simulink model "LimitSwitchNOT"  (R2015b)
settings: Solver=VariableStepAuto  StartTime=0.0  StopTime=10.0  RelTol=1e-3
libraries: vexarmcortexlib x4

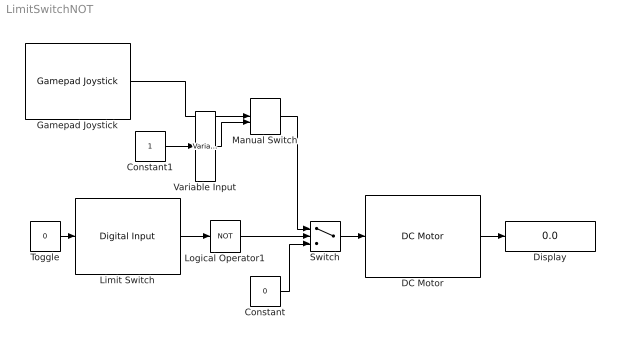
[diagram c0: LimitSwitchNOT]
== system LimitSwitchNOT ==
  Constant : Constant  Value=0
  Constant1 : Constant
  DC Motor : vexarmcortexlib/DC Motor  motor=5  scaleFactor=1/13.5  SimulationOut=on
  Display : Display
  Gamepad Joystick : vexarmcortexlib/Gamepad Joystick  joystick=1  chan=2  SimulationIn=on
  Limit Switch : vexarmcortexlib/Digital Input  inChan=1  SimulationIn=on
  Logical Operator1 : Logic  Operator=NOT  AllPortsSameDT=off  OutDataTypeStr=boolean
  Manual Switch : ManualSwitch  CurrentSetting=0
  Switch : Switch
  Toggle : Constant  Value=0
  Variable Input : vexarmcortexlib/Utilities/Variable Input  low=-127  gain=127  high=127
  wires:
  DC Motor/1 -> Display/1
  Switch/1 -> DC Motor/1
  Constant/1 -> Switch/3
  Manual Switch/1 -> Switch/1
  Variable Input/1 -> Manual Switch/2
  Constant1/1 -> Variable Input/1
  Gamepad Joystick/1 -> Manual Switch/1
  Toggle/1 -> Limit Switch/1
  Limit Switch/1 -> Logical Operator1/1
  Logical Operator1/1 -> Switch/2
